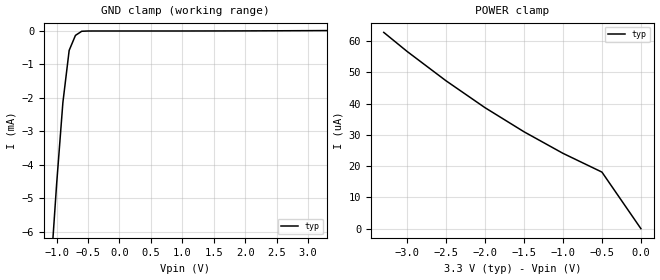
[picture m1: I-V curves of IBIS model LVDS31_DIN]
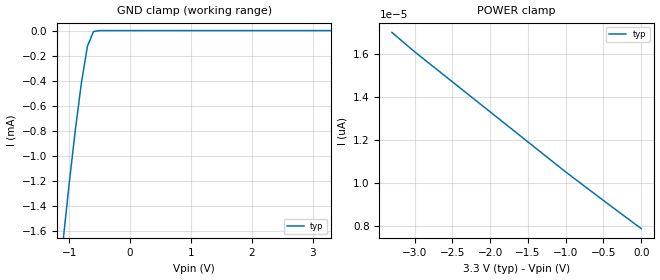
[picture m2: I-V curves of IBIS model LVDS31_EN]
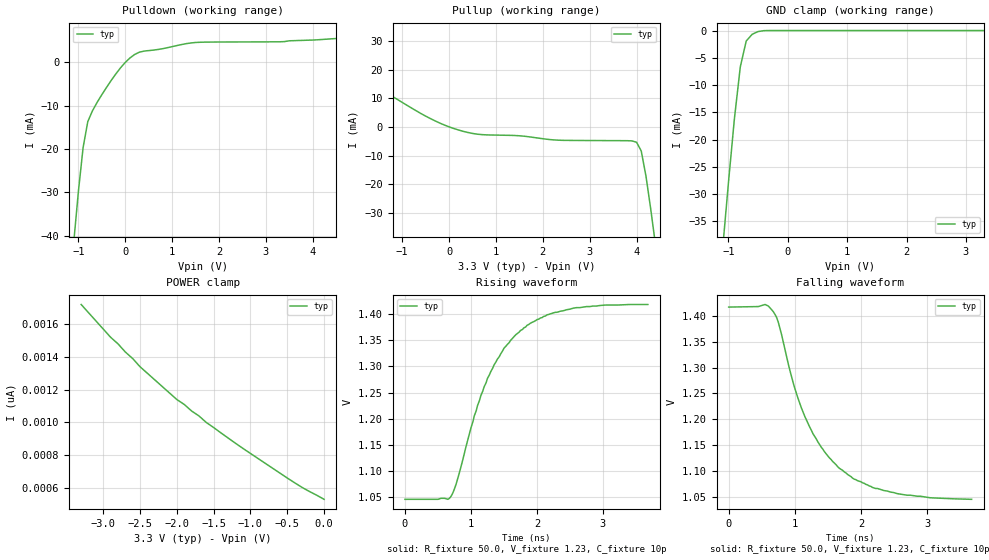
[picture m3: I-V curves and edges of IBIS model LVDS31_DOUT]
|   Texas Instruments Incorporated
|   Data Transmissions Products
|   IBIS Model for SN65LVDS31
|   16W Package
[IBIS Ver]   3.2
[Comment char]   |_char
[File name]   lvds31w.ibs
[File Rev]   3.0
[Date]   25Jul97   | Updated May 2009 for Ceramic W parasitics
[Source]   File originated at Texas Instruments Incorporated.
   Data Transmission Products Group. All data based on
   Bench Measurements.
[Notes]   Model revved in Nov02 to fix common-mode bug  -TMF-
[Disclaimer]
(C) Copyright Texas Instruments Incorporated 1997
   All rights reserved
  Texas Instruments Incorporated hereby grants the user of this IBIS
model a non-exclusive, nontransferable license to use this IBIS model
under the following terms.  Before using this IBIS model, the user
should read this license.  If the user does not accept these terms,
the IBIS model should be returned to Texas Instruments within 30 days.
  The user is granted this license only to use the IBIS model and
is not granted rights to sell, load, rent, lease or license the IBIS
model in whole or in part, or in modified form to anyone other than
user.  User may modify the IBIS model to suit its specific applications
but rights to derivative works and such modifications shall belong to
Texas Instruments.
  This IBIS model is provided on an "AS IS" basis and Texas Instruments
makes absolutely no warranty with respect to the information contained
herein.  TEXAS INSTRUMENTS DISCLAIMS AND CUSTOMER WAIVES ALL WARRANTIES,
EXPRESS OR IMPLIED, INCLUDING WARRANTIES OF MERCHANTABILITY OR FITNESS
FOR A PARTICULAR PURPOSE. The entire risk as to quality and performance
is with the Customer. ACCORDINGLY, IN NO EVENT SHALL THE COMPANY BE LIABLE
FOR ANY DAMAGES, WHETHER IN CONTRACT OR TORT,INCLUDING ANY LOST PROFITS
OR OTHER INCIDENTAL, CONSEQUENTIAL, EXEMPLARY, OR PUNITIVE DAMAGES ARISING
OUT OF THE USE OR APPLICATION OF THE IBIS model provided in this package.
Further, Texas Instruments reserves the right to discontinue or make changes
without notice to any product herein to improve reliability, function, or
design. Texas Instruments does not convey any license under patent rights
or any other intellectual property rights, including those of third parties.
Contact Texas Instruments at ATTN:DATA TRANSMISSIONS
[Copyright]   Copyright 1997, Texas Instruments, All Rights Reserved
[Component]   SN55LVDS31W
[Manufacturer]  Texas Instruments Incorporated
[Package]
|   typ   min   max
R_pkg   0.177   0.141   0.245
L_pkg   3.230nH   2.617nH   4.412nH
C_pkg   1.228pF   1.057pF   1.531pF
[Pin]   signal_name   model_name   R_pin   L_pin   C_pin
1   1A   LVDS31_DIN   0.244   4.385n   1.524p
2   1Y   LVDS31_DOUT   0.176   3.183n   1.235p
3   1Z   LVDS31_DOUT   0.142   2.637n   1.071p
4   G   LVDS31_EN   0.144   2.645n   1.060p
5   2Z   LVDS31_DOUT   0.147   2.708n   1.081p
6   2Y   LVDS31_DOUT   0.144   2.687n   1.092p
7   2A   LVDS31_DIN   0.176   3.182n   1.236p
8   GND   GND   0.245   4.412n   1.531p
9   3A   LVDS31_DIN   0.245   4.411n   1.531p
10   3Y   LVDS31_DOUT   0.176   3.183n   1.235p
11   3Z   LVDS31_DOUT   0.141   2.619n   1.064p
12   /G   LVDS31_EN   0.144   2.639n   1.057p
13   4Z   LVDS31_DOUT   0.150   2.772n   1.102p
14   4Y   LVDS31_DOUT   0.141   2.617n   1.063p
15   4A   LVDS31_DIN   0.176   3.182n   1.235p
16   VCC   POWER   0.245   4.411n   1.531p
[Diff_pin]   inv_pin   vdiff   tdelay_typ   tdelay_min   tdelay_max
| The 'xY' pin is Diff_pin and the 'xZ' pin is the inv_pin
2   3   NA   0 0 0
6   5   NA   0 0 0
10   11   NA   0 0 0
14   13   NA   0 0 0
| Models and submodels in the file (3): LVDS31_DIN (Input), LVDS31_EN (Input), LVDS31_DOUT (3-state)
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|   Driver Input  MODEL
[Model]   LVDS31_DIN
Model_type   Input
|Signals   1A,2A,3A,4A
Vinh = 2.0
Vinl = 0.8
|   typ   min   max
C_comp   1.0pF   NA   NA
|   typ   min   max
[Temperature Range]   25.0   NA   NA
[Voltage range]   3.3V   3.0V   3.6V
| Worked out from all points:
|   GND clamp passes 1 mA (typ) near -0.83 V on its own axis
[GND_clamp]
|   Voltage   I(typ)   I(min)   I(max)
-3.3V     -81mA      NA         NA
-1.1V     -7.36mA    NA         NA
-1V       -4.59mA    NA         NA
-900mV    -2.14mA    NA         NA
-800mV    -579uA     NA         NA
-700mV    -131uA     NA         NA
-600mV    -7.97uA    NA         NA
3.3V      12.9uA     NA         NA
[Power_clamp]
| Note that the[POWER_clamp]voltage table is referenced to Vcc
| and is calculated using Vtable=Vcc - Vmeasured.
|   Voltage   I(typ)   I(min)   I(max)
-3.3V     62.8uA     NA         NA
-3V       56.7uA     NA         NA
-2.5V     47.3uA     NA         NA
-2V       38.7uA     NA         NA
-1.5V     31uA       NA         NA
-1V       24.1uA     NA         NA
-500mV    18.1uA     NA         NA
0V        0A         NA         NA
|   Driver Enable  MODEL
[Model]   LVDS31_EN
Model_type   Input
|Signals   G,/G
Vinh = 2.0
Vinl = 0.8
|   typ   min   max
C_comp   1.0pF   NA   NA
|   typ   min   max
[Temperature Range]   25.0   NA   NA
[Voltage range]   3.3V   3.0V   3.6V
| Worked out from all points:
|   GND clamp passes 1 mA (typ) near -0.95 V on its own axis
[GND_clamp]
|   Voltage   I(typ)   I(min)   I(max)
-3.3V     -18.3mA    NA         NA
-1.1V     -1.69mA    NA         NA
-1V       -1.23mA    NA         NA
-900mV    -805uA     NA         NA
-800mV    -425uA     NA         NA
-700mV    -127uA     NA         NA
-600mV    -7.89uA    NA         NA
-500mV    -178nA     NA         NA
3.3V      7.86pA     NA         NA
[Power_clamp]
| Note that the[POWER_clamp]voltage table is referenced to Vcc
| and is calculated using Vtable=Vcc - Vmeasured.
|   Voltage   I(typ)   I(min)   I(max)
-3.3V     17pA       NA         NA
-3V       16.1pA     NA         NA
-2.5V     14.7pA     NA         NA
-2V       13.3pA     NA         NA
-1.5V     11.9pA     NA         NA
-1V       10.5pA     NA         NA
-500mV    9.17pA     NA         NA
0V        7.86pA     NA         NA
|   Driver Output  MODEL
[Model]   LVDS31_DOUT
Model_type   3-state
| Signals   1Y,1Z,2Y,2Z,3Y,3Z,4Y,4Z
Vmeas = 1.2V   |Reference voltage for timing measurements
Cref = 10pF   |Timing specification test load capacitance value
Rref = 50   |Note: 50 Ohm load; single ended configuration
Vref = 1.23V   |Timing specification test load voltage
| variable   typ   min   max
C_comp   1.0pF   NA   NA
|   typ   min   max
[Temperature Range]   25.0   NA   NA
[Voltage range]   3.3V   3.0V   3.6V
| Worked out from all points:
|   slope of the pulldown table from 0 to 0.495 V, typ, clamps not added: 182 ohm
|   slope of the pullup table from 0 to 0.495 V, typ, clamps not added: 216 ohm
|   GND clamp passes 1 mA (typ) near -0.63 V on its own axis
|   rising waveform, R_fixture 50.0, V_fixture 1.23, C_fixture 10p: 20-80 % time 692ps typ, NA min, NA max; typ from 1.04 V to 1.42 V
|   falling waveform, R_fixture 50.0, V_fixture 1.23, C_fixture 10p: 20-80 % time 728ps typ, NA min, NA max; typ from 1.42 V to 1.04 V
[Pulldown]
|   Voltage   I(typ)   I(min)   I(max)
-3.3V     -343mA     NA         NA
-1.1V     -41.6mA    NA         NA
-1V       -29.8mA    NA         NA
-900mV    -19.7mA    NA         NA
-800mV    -13.7mA    NA         NA
-600mV    -9.24mA    NA         NA
-200mV    -2.67mA    NA         NA
100mV     992uA      NA         NA
300mV     2.32mA     NA         NA
1.5V      4.56mA     NA         NA
4V        5.12mA     NA         NA
6.6V      7.6mA      NA         NA
[Pullup]
|   Voltage   I(typ)   I(min)   I(max)
| Note that the[Pullup]voltage table is referenced to Vcc
| and is calculated using Vtable=Vcc - Vmeasured.
-3.3V     35mA       NA         NA
-1.2V     10.6mA     NA         NA
-500mV    3.81mA     NA         NA
100mV     -516uA     NA         NA
700mV     -2.67mA    NA         NA
2.3V      -4.58mA    NA         NA
4V        -5.33mA    NA         NA
4.1V      -8.38mA    NA         NA
4.2V      -17.1mA    NA         NA
4.3V      -28.4mA    NA         NA
4.4V      -40.7mA    NA         NA
6.6V      -343mA     NA         NA
[GND_clamp]
|   Voltage   I(typ)   I(min)   I(max)
| Outputs in High Impedance (off)
-3.3V     -343mA     NA         NA
-1.1V     -40.4mA    NA         NA
-1V       -28mA      NA         NA
-900mV    -16.3mA    NA         NA
-800mV    -6.69mA    NA         NA
-700mV    -1.92mA    NA         NA
-600mV    -693uA     NA         NA
-500mV    -186uA     NA         NA
-300mV    -1.48uA    NA         NA
3.3V      531pA      NA         NA
[POWER_clamp]
|   Voltage   I(typ)   I(min)   I(max)
| Note that the [POWER_clamp] voltage table is referenced to Vcc
| and is calculated using Vtable = Vcc - Vmeasured.
| Outputs in Tri-state.
-3.3V     1.72nA     NA         NA
-2.9V     1.52nA     NA         NA
-2.8V     1.48nA     NA         NA
-2.5V     1.34nA     NA         NA
-2V       1.14nA     NA         NA
-1.9V     1.11nA     NA         NA
-1.6V     1nA        NA         NA
-1.1V     841pA      NA         NA
-400mV    632pA      NA         NA
0V        531pA      NA         NA
[Ramp]
| Note: Ramp rate measured on single-ended Driver Output.
|   typ   min   max
dV/dt_r   0.224/684ps   NA   NA
dV/dt_f   0.223/732ps   NA   NA
R_load = 50ohm | Note: These are single ended driver measurements
|   with 100ohm line-to-line termination and 4.5pF
|   line-to-ground capacitive load
[Rising Waveform]
R_fixture = 50.0
V_fixture = 1.23
C_fixture = 10p
L_fixture = 0n
|   V(typ)   V(min)   V(max)
0s        1.045V     NA         NA
700ps     1.051V     NA         NA
775ps     1.074V     NA         NA
1.05ns    1.205V     NA         NA
1.25ns    1.277V     NA         NA
1.5ns     1.335V     NA         NA
1.75ns    1.369V     NA         NA
2.15ns    1.399V     NA         NA
2.55ns    1.412V     NA         NA
3.68ns    1.419V     NA         NA
[Falling Waveform]
R_fixture = 50.0
V_fixture = 1.23
C_fixture = 10p
L_fixture = 0n
|   V(typ)   V(min)   V(max)
0s        1.417V     NA         NA
550ps     1.422V     NA         NA
675ps     1.408V     NA         NA
750ps     1.388V     NA         NA
975ps     1.271V     NA         NA
1.15ns    1.206V     NA         NA
1.4ns     1.146V     NA         NA
1.675ns   1.105V     NA         NA
2.45ns    1.059V     NA         NA
3.675ns   1.045V     NA         NA
